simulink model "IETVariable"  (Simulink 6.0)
settings: Solver=ode45  StartTime=0.0  StopTime=10  RelTol=1e-3
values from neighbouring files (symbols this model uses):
  b = S/Sm    (= 0.1)    [Constantes.m]    (also in ConstantesBck.m)
  beta = 0.95    [Constantes.m]    (also in ConstantesBck.m; ResCourV1.m = 1; ResCrV1.m = 1; ResEnerV1.m = 1)
  C = 1    [Constantes.m]    (also in ConstantesBck.m)
  Cdl = 603E-9    (= 6.03e-07)    [Constantes.m]    (also in ConstantesBck.m; ResCourV1.m = 7.313e-07; ResCrV1.m = 7.313e-07; ResEnerV1.m = 7.313e-07)
  Cmem = 1E-6*Sm*(1-b)    (= 2.826e-08)    [Constantes.m]    (also in ConstantesBck.m = 3.14e-11; ImpedanceZtissus.m = 4e-08; Ztissus.m = 4e-08; CalculCharge.m = 1)
  Fact = 10^2    (= 100)    [Constantes.m]    (also in ConstantesBck.m)
  gk = 36    [Constantes.m]    (also in ConstantesBck.m; sim_hh.m)
  gl = 0.3    [Constantes.m]    (also in ConstantesBck.m; sim_hh.m)
  gna = 120    [Constantes.m]    (also in ConstantesBck.m; sim_hh.m)
  h0 = 0.5961    [Constantes.m]    (also in ConstantesBck.m)
  m0 = 0.0529    [Constantes.m]    (also in ConstantesBck.m)
  mK = 0    [Constantes.m]    (also in ConstantesBck.m)
  mL = 0    [Constantes.m]    (also in ConstantesBck.m)
  mNa = 0    [Constantes.m]    (also in ConstantesBck.m)
  n0 = 0.3177    [Constantes.m]    (also in ConstantesBck.m)
  rapportIE = 10    [Constantes.m]
  Rcan = 6.398E3*Sm*(1-b)    (= 180.80748)    [Constantes.m]    (also in ConstantesBck.m = 0.03454; ImpedanceZtissus.m = 44; Ztissus.m = 44)
  Rct = 185.6E3    (= 185600)    [Constantes.m]    (also in ConstantesBck.m; ResCourV1.m = 605200; ResCrV1.m = 605200; ResEnerV1.m = 605200)
  Rext = 2.9E3    (= 2900)    [Constantes.m]    (also in ConstantesBck.m)
  Rint = 2.9E2    (= 290)    [Constantes.m]    (also in ConstantesBck.m = 400)
  sigma = 66466    [Constantes.m]    (also in ConstantesBck.m; ResCourV1.m = 68000; ResCrV1.m = 68000; ResEnerV1.m = 68000)
  Sm = 3.14e-2    (= 0.0314)    [Constantes.m]    (also in ConstantesBck.m = 0.000314)
  Vk = -82    [Constantes.m]    (also in ConstantesBck.m)
  Vl = -59    [Constantes.m]    (also in ConstantesBck.m)
  Vna = 45    [Constantes.m]    (also in ConstantesBck.m)
  Vr = -70    [Constantes.m]    (also in ConstantesBck.m)
undefined symbols (not defined in the file or in its folder): ln
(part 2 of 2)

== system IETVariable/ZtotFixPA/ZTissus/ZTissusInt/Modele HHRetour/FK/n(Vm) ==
  note: V
  note: alpha_*(1-n)
  note: beta_n*n
  note: n
  note: n
  Vm : Inport  Port=1  LatchInput=off
  (1-n) : Fcn  Expr=1-u
  Integrator1 : Integrator  InitialCondition=n0
  Product : Product
  Product1 : Product
  Sum1 : Sum  Inputs=+-
  V : Fcn  Expr=u-Vr
  alpha_n : Fcn  Expr=(0.01*(10-u))/(exp((10-u)/10)-1)
  beta_n : Fcn  Expr=0.125*exp(-u/80)
  n : Outport  InitialOutput=0
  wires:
  V/1 -> alpha_n/1, beta_n/1
  alpha_n/1 -> Product/2
  (1-n)/1 -> Product/1
  beta_n/1 -> Product1/1
  Product/1 -> Sum1/1
  Product1/1 -> Sum1/2
  Sum1/1 -> Integrator1/1
  Integrator1/1 -> (1-n)/1, Product1/2, n/1
  Vm/1 -> V/1

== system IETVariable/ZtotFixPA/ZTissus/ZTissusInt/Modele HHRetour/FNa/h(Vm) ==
  note: h
  note: h
  note: beta_h*h
  note: alpha_h*(1-h)
  note: V
  Vm : Inport  Port=1  LatchInput=off
  (1-h) : Fcn  Expr=1-u
  Integrator1 : Integrator  InitialCondition=h0
  Product : Product
  Product1 : Product
  Sum1 : Sum  Inputs=+-
  V : Fcn  Expr=u-Vr
  alpha_h : Fcn  Expr=0.07*exp(-u/20)
  beta_h : Fcn  Expr=1/(exp((30-u)/10)+1)
  h : Outport  InitialOutput=0
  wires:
  Vm/1 -> V/1
  Integrator1/1 -> h/1, Product1/2, (1-h)/1
  Sum1/1 -> Integrator1/1
  Product1/1 -> Sum1/2
  Product/1 -> Sum1/1
  beta_h/1 -> Product1/1
  (1-h)/1 -> Product/1
  alpha_h/1 -> Product/2
  V/1 -> beta_h/1, alpha_h/1

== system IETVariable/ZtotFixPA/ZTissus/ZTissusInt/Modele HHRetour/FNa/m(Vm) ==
  note: m
  note: m
  note: beta_m*m
  note: alpha_m*(1-m)
  note: V
  Vm : Inport  Port=1  LatchInput=off
  (1-m) : Fcn  Expr=1-u
  Integrator1 : Integrator  InitialCondition=m0
  Product : Product
  Product1 : Product
  Sum1 : Sum  Inputs=+-
  V : Fcn  Expr=u-Vr
  alpha_m : Fcn  Expr=(0.1*(25-u))/(exp((25-u)/10)-1)
  beta_m : Fcn  Expr=4*exp(-u/18)
  n : Outport  InitialOutput=0
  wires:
  Vm/1 -> V/1
  Integrator1/1 -> n/1, Product1/2, (1-m)/1
  Sum1/1 -> Integrator1/1
  Product1/1 -> Sum1/2
  Product/1 -> Sum1/1
  beta_m/1 -> Product1/1
  (1-m)/1 -> Product/1
  alpha_m/1 -> Product/2
  V/1 -> beta_m/1, alpha_m/1

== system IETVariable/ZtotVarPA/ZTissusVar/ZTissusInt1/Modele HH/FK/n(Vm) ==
  note: V
  note: alpha_*(1-n)
  note: beta_n*n
  note: n
  note: n
  Vm : Inport  Port=1  LatchInput=off
  (1-n) : Fcn  Expr=1-u
  Integrator1 : Integrator  InitialCondition=n0
  Product : Product
  Product1 : Product
  Sum1 : Sum  Inputs=+-
  V : Fcn  Expr=u-Vr
  alpha_n : Fcn  Expr=(0.01*(10-u))/(exp((10-u)/10)-1)
  beta_n : Fcn  Expr=0.125*exp(-u/80)
  n : Outport  InitialOutput=0
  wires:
  V/1 -> alpha_n/1, beta_n/1
  alpha_n/1 -> Product/2
  (1-n)/1 -> Product/1
  beta_n/1 -> Product1/1
  Product/1 -> Sum1/1
  Product1/1 -> Sum1/2
  Sum1/1 -> Integrator1/1
  Integrator1/1 -> (1-n)/1, Product1/2, n/1
  Vm/1 -> V/1

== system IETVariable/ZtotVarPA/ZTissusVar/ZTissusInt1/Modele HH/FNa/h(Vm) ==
  note: h
  note: h
  note: beta_h*h
  note: alpha_h*(1-h)
  note: V
  Vm : Inport  Port=1  LatchInput=off
  (1-h) : Fcn  Expr=1-u
  Integrator1 : Integrator  InitialCondition=h0
  Product : Product
  Product1 : Product
  Sum1 : Sum  Inputs=+-
  V : Fcn  Expr=u-Vr
  alpha_h : Fcn  Expr=0.07*exp(-u/20)
  beta_h : Fcn  Expr=1/(exp((30-u)/10)+1)
  h : Outport  InitialOutput=0
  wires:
  Vm/1 -> V/1
  Integrator1/1 -> h/1, Product1/2, (1-h)/1
  Sum1/1 -> Integrator1/1
  Product1/1 -> Sum1/2
  Product/1 -> Sum1/1
  beta_h/1 -> Product1/1
  (1-h)/1 -> Product/1
  alpha_h/1 -> Product/2
  V/1 -> beta_h/1, alpha_h/1

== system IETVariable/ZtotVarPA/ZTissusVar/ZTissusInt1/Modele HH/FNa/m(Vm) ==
  note: m
  note: m
  note: beta_m*m
  note: alpha_m*(1-m)
  note: V
  Vm : Inport  Port=1  LatchInput=off
  (1-m) : Fcn  Expr=1-u
  Integrator1 : Integrator  InitialCondition=m0
  Product : Product
  Product1 : Product
  Sum1 : Sum  Inputs=+-
  V : Fcn  Expr=u-Vr
  alpha_m : Fcn  Expr=(0.1*(25-u))/(exp((25-u)/10)-1)
  beta_m : Fcn  Expr=4*exp(-u/18)
  n : Outport  InitialOutput=0
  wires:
  Vm/1 -> V/1
  Integrator1/1 -> n/1, Product1/2, (1-m)/1
  Sum1/1 -> Integrator1/1
  Product1/1 -> Sum1/2
  Product/1 -> Sum1/1
  beta_m/1 -> Product1/1
  (1-m)/1 -> Product/1
  alpha_m/1 -> Product/2
  V/1 -> beta_m/1, alpha_m/1

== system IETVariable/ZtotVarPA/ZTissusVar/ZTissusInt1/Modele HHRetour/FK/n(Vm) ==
  note: V
  note: alpha_*(1-n)
  note: beta_n*n
  note: n
  note: n
  Vm : Inport  Port=1  LatchInput=off
  (1-n) : Fcn  Expr=1-u
  Integrator1 : Integrator  InitialCondition=n0
  Product : Product
  Product1 : Product
  Sum1 : Sum  Inputs=+-
  V : Fcn  Expr=u-Vr
  alpha_n : Fcn  Expr=(0.01*(10-u))/(exp((10-u)/10)-1)
  beta_n : Fcn  Expr=0.125*exp(-u/80)
  n : Outport  InitialOutput=0
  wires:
  V/1 -> alpha_n/1, beta_n/1
  alpha_n/1 -> Product/2
  (1-n)/1 -> Product/1
  beta_n/1 -> Product1/1
  Product/1 -> Sum1/1
  Product1/1 -> Sum1/2
  Sum1/1 -> Integrator1/1
  Integrator1/1 -> (1-n)/1, Product1/2, n/1
  Vm/1 -> V/1

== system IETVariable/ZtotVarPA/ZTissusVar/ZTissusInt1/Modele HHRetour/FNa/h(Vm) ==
  note: h
  note: h
  note: beta_h*h
  note: alpha_h*(1-h)
  note: V
  Vm : Inport  Port=1  LatchInput=off
  (1-h) : Fcn  Expr=1-u
  Integrator1 : Integrator  InitialCondition=h0
  Product : Product
  Product1 : Product
  Sum1 : Sum  Inputs=+-
  V : Fcn  Expr=u-Vr
  alpha_h : Fcn  Expr=0.07*exp(-u/20)
  beta_h : Fcn  Expr=1/(exp((30-u)/10)+1)
  h : Outport  InitialOutput=0
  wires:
  Vm/1 -> V/1
  Integrator1/1 -> h/1, Product1/2, (1-h)/1
  Sum1/1 -> Integrator1/1
  Product1/1 -> Sum1/2
  Product/1 -> Sum1/1
  beta_h/1 -> Product1/1
  (1-h)/1 -> Product/1
  alpha_h/1 -> Product/2
  V/1 -> beta_h/1, alpha_h/1

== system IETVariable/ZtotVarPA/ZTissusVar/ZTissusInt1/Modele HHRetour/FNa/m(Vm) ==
  note: m
  note: m
  note: beta_m*m
  note: alpha_m*(1-m)
  note: V
  Vm : Inport  Port=1  LatchInput=off
  (1-m) : Fcn  Expr=1-u
  Integrator1 : Integrator  InitialCondition=m0
  Product : Product
  Product1 : Product
  Sum1 : Sum  Inputs=+-
  V : Fcn  Expr=u-Vr
  alpha_m : Fcn  Expr=(0.1*(25-u))/(exp((25-u)/10)-1)
  beta_m : Fcn  Expr=4*exp(-u/18)
  n : Outport  InitialOutput=0
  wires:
  Vm/1 -> V/1
  Integrator1/1 -> n/1, Product1/2, (1-m)/1
  Sum1/1 -> Integrator1/1
  Product1/1 -> Sum1/2
  Product/1 -> Sum1/1
  beta_m/1 -> Product1/1
  (1-m)/1 -> Product/1
  alpha_m/1 -> Product/2
  V/1 -> beta_m/1, alpha_m/1

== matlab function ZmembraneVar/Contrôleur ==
function [y,temp] = fcn(u,calc)
% This block supports an embeddable subset of the MATLAB language.
% See the help menu for details. 

if u == 0
    y = 0;
    temp = 1E-6;
else
    y = calc;
    temp = u;
end

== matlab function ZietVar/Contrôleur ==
function [y,temp] = fcn(u,calc)
% This block supports an embeddable subset of the MATLAB language.
% See the help menu for details. 

if u == 0
    y = 0;
    temp = 1E-6;
else
    y = calc;
    temp = u;
end

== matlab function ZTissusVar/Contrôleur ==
function [y,temp] = fcn(u,calc)
% This block supports an embeddable subset of the MATLAB language.
% See the help menu for details. 

if u == 0
    y = 0;
    temp = 1E-6;
else
    y = calc;
    temp = u;
end

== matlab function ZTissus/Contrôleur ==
function [y,temp] = fcn(u,calc)
% This block supports an embeddable subset of the MATLAB language.
% See the help menu for details. 

if u == 0
    y = 0;
    temp = 1E-6;
else
    y = calc;
    temp = u;
end

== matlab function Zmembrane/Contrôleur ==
function [y,temp] = fcn(u,calc)
% This block supports an embeddable subset of the MATLAB language.
% See the help menu for details. 

if u == 0
    y = 0;
    temp = 1E-6;
else
    y = calc;
    temp = u;
end

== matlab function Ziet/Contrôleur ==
function [y,temp] = fcn(u,calc)
% This block supports an embeddable subset of the MATLAB language.
% See the help menu for details. 

if u == 0
    y = 0;
    temp = 1E-6;
else
    y = calc;
    temp = u;
end

== matlab function ZtotFixNPA
/Ziet/Contrôleur ==
function [y,temp] = fcn(u,calc)
% This block supports an embeddable subset of the MATLAB language.
% See the help menu for details. 

if u == 0
    y = 0;
    temp = 1E-6;
else
    y = calc;
    temp = u;
end

== matlab function ZtotFixNPA
/Zmembrane/Contrôleur ==
function [y,temp] = fcn(u,calc)
% This block supports an embeddable subset of the MATLAB language.
% See the help menu for details. 

if u == 0
    y = 0;
    temp = 1E-6;
else
    y = calc;
    temp = u;
end

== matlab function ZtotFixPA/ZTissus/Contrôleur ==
function [y,temp] = fcn(u,calc)
% This block supports an embeddable subset of the MATLAB language.
% See the help menu for details. 

if u == 0
    y = 0;
    temp = 1E-6;
else
    y = calc;
    temp = u;
end

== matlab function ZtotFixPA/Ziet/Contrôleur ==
function [y,temp] = fcn(u,calc)
% This block supports an embeddable subset of the MATLAB language.
% See the help menu for details. 

if u == 0
    y = 0;
    temp = 1E-6;
else
    y = calc;
    temp = u;
end

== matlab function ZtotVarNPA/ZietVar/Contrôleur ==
function [y,temp] = fcn(u,calc)
% This block supports an embeddable subset of the MATLAB language.
% See the help menu for details. 

if u == 0
    y = 0;
    temp = 1E-6;
else
    y = calc;
    temp = u;
end

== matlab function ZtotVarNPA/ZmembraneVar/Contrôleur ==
function [y,temp] = fcn(u,calc)
% This block supports an embeddable subset of the MATLAB language.
% See the help menu for details. 

if u == 0
    y = 0;
    temp = 1E-6;
else
    y = calc;
    temp = u;
end

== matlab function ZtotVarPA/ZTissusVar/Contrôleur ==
function [y,temp] = fcn(u,calc)
% This block supports an embeddable subset of the MATLAB language.
% See the help menu for details. 

if u == 0
    y = 0;
    temp = 1E-6;
else
    y = calc;
    temp = u;
end

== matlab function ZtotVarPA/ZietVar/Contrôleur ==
function [y,temp] = fcn(u,calc)
% This block supports an embeddable subset of the MATLAB language.
% See the help menu for details. 

if u == 0
    y = 0;
    temp = 1E-6;
else
    y = calc;
    temp = u;
end
